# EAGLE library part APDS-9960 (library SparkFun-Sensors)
Avago APDS-9960 Digital Proximity, Ambient Light, RGB, and Gesture Sensor. The APDS-9960 offers ambient light and color measuring, proximity detection, and touchless gesture sensing. It features UV and IR blocking filters, four separate diodes sensitive to different directions, and an I2C compatible interface. Datasheet SparkFun Products SparkFun RGB and Gesture Sensor - APDS-9960 (SEN-12787)
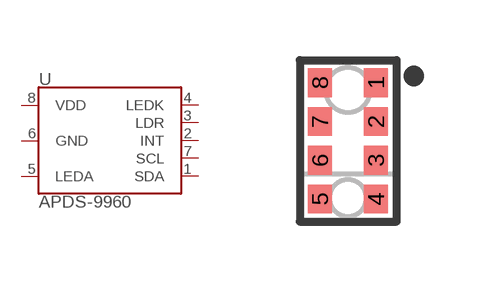
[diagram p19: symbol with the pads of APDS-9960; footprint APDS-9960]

Designator prefix U

## APDS-9960 (PROD_ID: SEN-12005)  [APDS-9960]
1  SDA
2  INT
3  LDR
4  LEDK
5  LEDA
6  GND
7  SCL
8  VDD

## Footprint APDS-9960 (pad centres in mm)
APDS-9960 Proximity, Light, RGB, Gesture Sensor Datasheet Specifications: Pin Count: 8 Dimensions: 3.94 x 2.36 x 1.35 mm Pitch: 0.97 mm Devices Using: APDS-9960
smd 0.6 x 0.72: 1 0.7,1.455; 2 0.7,0.485; 3 0.7,-0.485; 4 0.7,-1.455; 5 -0.7,-1.455; 6 -0.7,-0.485; 7 -0.7,0.485; 8 -0.7,1.455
